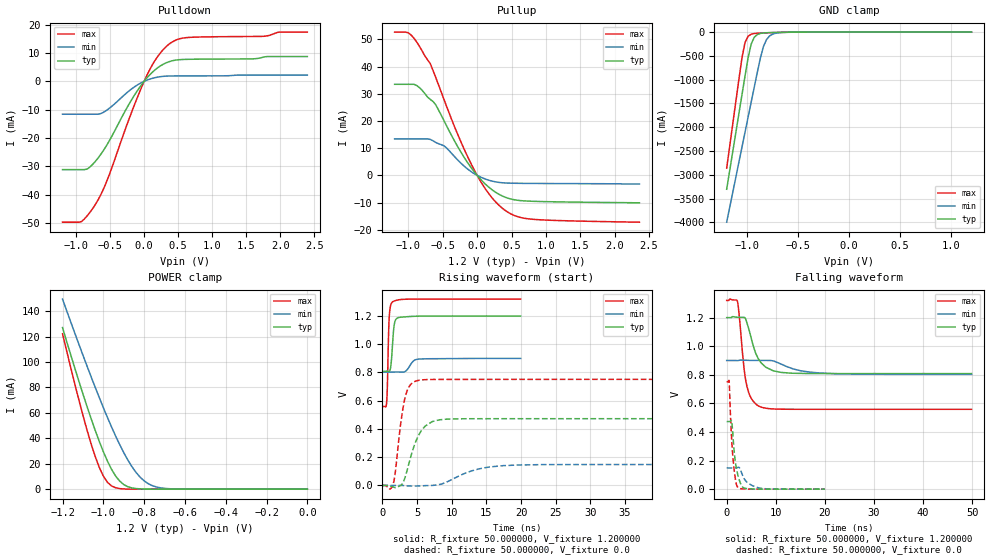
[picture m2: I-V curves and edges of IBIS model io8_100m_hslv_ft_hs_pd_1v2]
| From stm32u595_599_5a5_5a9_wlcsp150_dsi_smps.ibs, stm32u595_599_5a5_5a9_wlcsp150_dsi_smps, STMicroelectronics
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|   Model io8_100m_hslv_ft_hs_pd_1v2
[Model]  io8_100m_hslv_ft_hs_pd_1v2
Model_type I/O
Polarity   Non-Inverting
Enable   Active-Low
Vinl =   0.360000V
Vinh =   0.840000V
Vmeas =  0.600000V
Cref =   50.000000pF
Rref =   100.000000M
Vref =   0.0V
C_comp   3.030100pF   2.960800pF   3.078300pF
[Temperature Range]   25.000000   0.140000k   -40.000000
[Pullup Reference]   1.200000V   0.900000V   1.320000V
[Pulldown Reference]   0.0V   0.0V   0.0V
[POWER Clamp Reference]   1.200000V   0.900000V   1.320000V
[GND Clamp Reference]   0.0V   0.0V   0.0V
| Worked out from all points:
|   slope of the pulldown table from 0 to 0.18 V, typ, clamps not added: 40.7 ohm
|   slope of the pullup table from 0 to 0.18 V, typ, clamps not added: 39.5 ohm
|   GND clamp passes 1 mA (typ) near -0.51 V on its own axis
|   POWER clamp passes 1 mA (typ) near -0.86 V on its own axis
|   rising waveform, R_fixture 50.000000, V_fixture 1.200000: 20-80 % time 362ps typ, 843ps min, 238ps max; typ from 0.808 V to 1.2 V
|   rising waveform, R_fixture 50.000000, V_fixture 0.0: 20-80 % time 2ns typ, 4.56ns min, 1.18ns max; typ from 0 V to 0.472 V
|   falling waveform, R_fixture 50.000000, V_fixture 1.200000: 20-80 % time 2.46ns typ, 5.46ns min, 1.5ns max; typ from 1.2 V to 0.808 V
|   falling waveform, R_fixture 50.000000, V_fixture 0.0: 20-80 % time 1.05ns typ, 1.99ns min, 803ps max; typ from 0.472 V to 0 V
[Pulldown]
|Voltage   I(typ)   I(min)   I(max)
-1.2V     -31.16mA   -11.61mA   -49.71mA
-920mV    -31.16mA   -11.61mA   -49.48mA
-840mV    -31mA      -11.61mA   -47.54mA
-720mV    -28.33mA   -11.61mA   -43.58mA
-560mV    -22.95mA   -10.37mA   -35.89mA
-200mV    -7.146mA   -2.964mA   -11.89mA
0V        0A         -1pA       0A
160mV     4.047mA    1.298mA    7.361mA
360mV     6.87mA     1.87mA     13mA
640mV     7.765mA    1.923mA    15.46mA
1.76V     8.564mA    2.187mA    15.9mA
2.4V      8.742mA    2.187mA    17.38mA
[Pullup]
|Voltage   I(typ)   I(min)   I(max)
-1.2V     33.49mA    13.42mA    52.68mA
-960mV    33.49mA    13.42mA    51.61mA
-840mV    32.28mA    13.42mA    47.51mA
-680mV    27.9mA     13.19mA    41.05mA
-600mV    25.88mA    12.07mA    35.87mA
-480mV    20.01mA    10.83mA    27.79mA
-280mV    10.44mA    5.592mA    14.93mA
-80mV     2.58mA     1.232mA    3.849mA
160mV     -4.145mA   -1.713mA   -6.415mA
400mV     -7.962mA   -2.792mA   -12.75mA
800mV     -9.537mA   -2.973mA   -16.14mA
2.36V     -10.1mA    -3.2mA     -17.23mA
[GND_clamp]
|Voltage   I(typ)   I(min)   I(max)
-1.2V     -3.305A    -3.998A    -2.862A
-1.05V    -1.316A    -2.418A    -539.3mA
-1.02V    -921mA     -2.103A    -218.8mA
-990mV    -539.5mA   -1.788A    -87.45mA
-960mV    -252.2mA   -1.474A    -44.37mA
-930mV    -110.5mA   -1.16A     -30.33mA
-870mV    -28.04mA   -549.1mA   -21.1mA
-840mV    -18.44mA   -305.6mA   -18.29mA
-810mV    -13.92mA   -159.7mA   -15.75mA
-780mV    -11.24mA   -82.36mA   -13.39mA
-600mV    -2.986mA   -4.279mA   -3.072mA
1.2V      30.28uA    18.17uA    37.27uA
[POWER_clamp]
|Voltage   I(typ)   I(min)   I(max)
-1.2V     127mA      149.4mA    122.2mA
-1.12V    84.97mA    114mA      70.27mA
-1.06V    55.51mA    88.42mA    35.67mA
-1.02V    37.63mA    72.04mA    17.17mA
-1V       29.51mA    64.13mA    10.3mA
-960mV    15.69mA    48.99mA    2.571mA
-900mV    3.624mA    28.77mA    182.8uA
-840mV    490.7uA    13.24mA    11.35uA
-800mV    116.8uA    6.532mA    1.77uA
-740mV    13.2uA     1.723mA    109.1nA
-620mV    167.3nA    79.35uA    0A
0V        0A         17.84nA    0A
[Ramp]
| variable   typ   min   max
dV/dt_r  0.28340/1.99687n   88.81788m/4.55232n  0.45044/1.18302n
dV/dt_f  0.23486/2.45254n   58.03200m/5.45559n  0.45673/1.50159n
R_load = 50.000000
[Rising Waveform]
R_fixture= 50.000000
V_fixture= 1.200000
V_fixture_min= 0.900000
V_fixture_max= 1.320000
|time   V(typ)   V(min)   V(max)
0s        808mV      802.7mV    558.3mV
600.6ps   808.7mV    802.7mV    579.2mV
720.7ps   808.6mV    802.7mV    698.5mV
880.9ps   807.1mV    802.7mV    1.046V
1.001ns   805.7mV    802.7mV    1.2V
1.481ns   1.009V     802.8mV    1.3V
1.802ns   1.158V     802.9mV    1.307V
2.442ns   1.19V      802.8mV    1.315V
5.165ns   1.198V     893.9mV    1.319V
19.94ns   1.199V     899.4mV    1.319V
[Rising Waveform]
R_fixture= 50.000000
V_fixture= 0.0
V_fixture_min= 0.0
V_fixture_max= 0.0
|time   V(typ)   V(min)   V(max)
0s        -14.65uV   -6.115uV   -48.7uV
1.502ns   -10.14mV   -40.8uV    -1.013mV
1.802ns   -14.87mV   -38.23uV   69.37mV
3.203ns   45.81mV    -1.916mV   606.2mV
3.904ns   168.6mV    -3.803mV   703mV
4.905ns   320.8mV    -4.272mV   740mV
6.206ns   421.2mV    -1.571mV   748.8mV
9.009ns   468.4mV    18.4mV     750.7mV
17.52ns   472.4mV    140.2mV    750.9mV
49.85ns   472.4mV    148.1mV    750.9mV
[Falling Waveform]
R_fixture= 50.000000
V_fixture= 1.200000
V_fixture_min= 0.900000
V_fixture_max= 1.320000
|time   V(typ)   V(min)   V(max)
0s        1.199V     899.4mV    1.319V
2.202ns   1.202V     899.1mV    1.313V
3.504ns   1.201V     901.4mV    854.1mV
4.104ns   1.164V     900.9mV    721.8mV
5.105ns   1.04V      900.1mV    629.1mV
6.707ns   898.1mV    899.9mV    577.7mV
9.409ns   828.5mV    896.6mV    560.9mV
13.11ns   810.7mV    845.8mV    558.5mV
21.92ns   808mV      807mV      558.3mV
49.85ns   808mV      802.7mV    558.3mV
[Falling Waveform]
R_fixture= 50.000000
V_fixture= 0.0
V_fixture_min= 0.0
V_fixture_max= 0.0
|time   V(typ)   V(min)   V(max)
0s        472.4mV    148.1mV    750.9mV
480.5ps   472.6mV    148.2mV    756.6mV
1.001ns   478.8mV    148.2mV    357mV
1.281ns   369.4mV    148.2mV    218.2mV
1.642ns   224.7mV    148.1mV    102.8mV
1.962ns   148.8mV    148.6mV    36.24mV
2.322ns   93.06mV    152.4mV    9.961mV
3.403ns   9.8mV      83.14mV    1.606mV
6.406ns   695.3uV    10.18mV    73.86uV
19.94ns   -14.65uV   -6.115uV   -48.7uV
